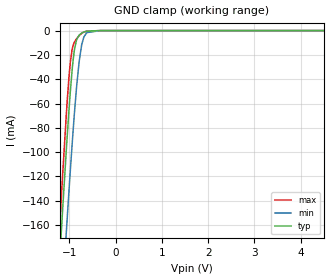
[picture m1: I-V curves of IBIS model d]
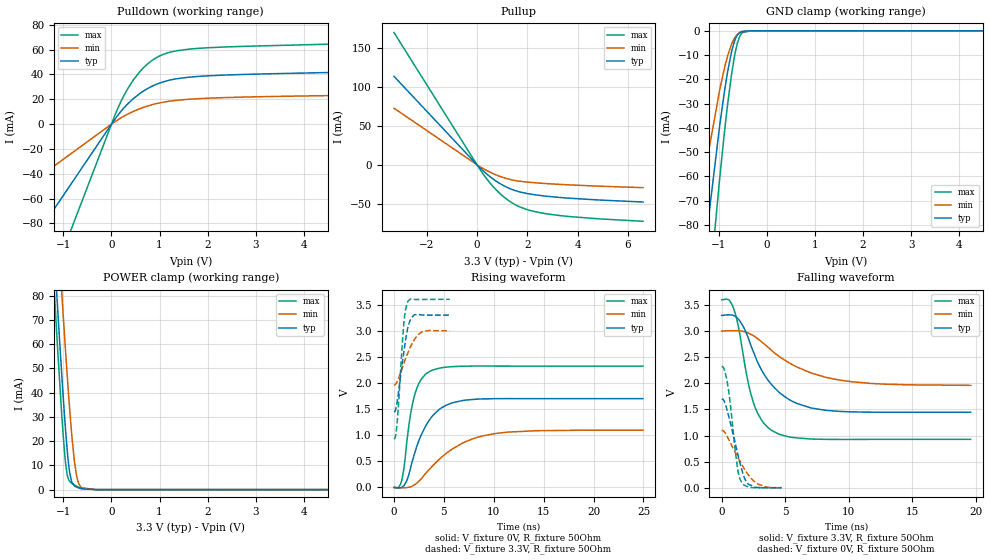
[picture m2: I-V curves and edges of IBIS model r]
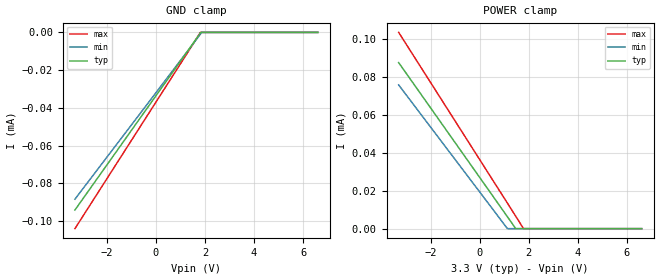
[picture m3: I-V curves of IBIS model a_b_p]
|Texas Instruments Incorporated
| 3.3V-supply RS-485
| Marketing part#   Digital Voltage Range   Package-type   #pins
| SN65HVD77DGK   3.0V-3.6V   VSSOP   8
| SN65HVD77DGKR   3.0V-3.6V   VSSOP   8
| SN65HVD77D   3.0V-3.6V   SOIC   8
| SN65HVD77DR   3.0V-3.6V   SOIC   8
[IBIS Ver]   4.1
[File name]   sn65hvd77.ibs
[File Rev]   1.0
[Date]   7/9/2014
[Source]
| Texas Instruments Incorporated.
| Analog-eLab Design Center, HPA
| 12500 TI Blvd
| Dallas, TX -75243
[Notes]   Revision History:
| Rev 1.0: 7/9/2014
| - Initial version of the model
| - Model generated from simulations in TISPICE
| - Model matched to SPICE simulation
| - C_comp although listed in numerical order of value are
|   obtained from varying PVT conditions. For PVT conditions for
|   each specific value refer the buffer description under
|   respective [Model]. IBIS model user is responsible for using
|   appropriate C_comp to simulate for Signal Integrity.
|* EXCEPTION:   *
|* - For model d, there is leakage current in the GND   *
|*   clamp I-V Table because of the pullup on pad.   *
|* - For models a_b_p and a_b_n, there is leakage current in the   *
|*   POWER clamp and GND clamp I-V Table because of the resistor   *
|*   network connected to pad.   *
[Disclaimer]
| This model is designed as an aid for customers of Texas Instruments.
| TI and its licensors and suppliers make no warranties, either expressed
| or implied, with respect to this  model, including the warranties of
| merchantability or fitness for a particular purpose. The model is
| provided solely on an "as is" basis. The entire risk as to its quality
| and performance is with the customer.
[Copyright]
(C) Copyright 2014 Texas Instruments Incorporated.All rights reserved.
|   SN65HVD77DGK
[Component]   SN65HVD77DGK
[Manufacturer]   TI
[Package]   |8 VSSOP  -  DGK package
|   typ   min   max
R_pkg   0.2   0.16   0.24
L_pkg   1.5nH   1.2nH   1.8nH
C_pkg   0.4pF   0.32pF   0.48pF
[Pin]  signal_name   model_name   R_pin   L_pin   C_pin
1   VCC   power   NA   NA   NA
2   R   r   NA   NA   NA
3   D   d   NA   NA   NA
4   GND   gnd   NA   NA   NA
5   Y   y_z_p   NA   NA   NA
6   Z   y_z_n   NA   NA   NA
7   B   a_b_n   NA   NA   NA
8   A   a_b_p   NA   NA   NA
[Diff_pin]   inv_pin   vdiff   tdelay_typ   tdelay_min   tdelay_max
5   6   0   NA   NA   NA
8   7   0.2V   NA   NA   NA
|   SN65HVD77D
[Component]   SN65HVD77D
[Manufacturer]   TI
[Package]   |8 SOIC  -  D package
|   typ   min   max
R_pkg   0.2   0.16   0.24
L_pkg   1.5nH   1.2nH   1.8nH
C_pkg   0.4pF   0.32pF   0.48pF
[Pin]  signal_name   model_name   R_pin   L_pin   C_pin
1   VCC   power   NA   NA   NA
2   R   r   NA   NA   NA
3   D   d   NA   NA   NA
4   GND   gnd   NA   NA   NA
5   Y   y_z_p   NA   NA   NA
6   Z   y_z_n   NA   NA   NA
7   B   a_b_n   NA   NA   NA
8   A   a_b_p   NA   NA   NA
[Diff_pin]   inv_pin   vdiff   tdelay_typ   tdelay_min   tdelay_max
5   6   0   NA   NA   NA
8   7   0.2V   NA   NA   NA
| Models and submodels in the file (6): d (Input), r (3-state), a_b_p (Input), a_b_n (Input), y_z_p (Output), y_z_n (Output)
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|   d Model
[Model]   d
Model_type   Input
Vinl = 0.8
Vinh = 2
|   typ   min   max
|   (nom PVT)   (fast PVT)   (slow PVT)
|Average
C_comp   2.191e-12   2.010e-12   2.367e-12
| Where nom  PVT is Nominal Process, 3.3V, 27C
|   Fast PVT is Strong Process,  3.6V, -40C
|   Slow PVT is Weak Process,   3V, 150C
[Voltage Range]   3.3   3   3.6
|Ambient Temperature   25   125   -40
|Junction Temperature
[Temperature Range]   27   150   -40
[Power Clamp Reference]   3.3   3   3.6
[GND Clamp Reference]   0   0   0
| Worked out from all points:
|   GND clamp passes 1 mA (typ) near -0.67 V on its own axis
[GND Clamp]
|   Voltage   I(typ)   I(min)   I(max)
-3.3V     -1.706A    -1.709A    -1.74A
-1.33V    -268.5mA   -332.2mA   -244.5mA
-1.176V   -166.3mA   -233.3mA   -138.2mA
-1.064V   -96.82mA   -164.4mA   -67.68mA
-980.1mV  -50.33mA   -115.2mA   -26.33mA
-945.6mV  -34.42mA   -96.08mA   -16.53mA
-891mV    -15.86mA   -67.76mA   -9.449mA
-789mV    -3.689mA   -25.45mA   -4.166mA
-735mV    -2.045mA   -11.84mA   -2.349mA
-686.4mV  -1.145mA   -5.17mA    -1.213mA
-330mV    -2.214uA   -10.64uA   -3.071uA
6.6V      0A         0A         0A
[POWER Clamp]
|   Voltage   I(typ)   I(min)   I(max)
-3.3V     0A         0A         0A
0V        0A         0A         0A
6.6V      0A         0A         0A
|   r Model
[Model]   r
Model_type   3-state
Polarity   Non-Inverting
Vmeas = 1.65
Vref = 0
Cref = 2pF
Rref = 100
|   typ   min   max
|   (nom PVT)   (fast PVT)   (slow PVT)
C_comp   1.738e-12   1.292e-12   1.903e-12
| Where nom  PVT is Nominal Process, 3.3V, 27C
|   Fast PVT is Strong Process,  3.6V, -40C
|   Slow PVT is Weak Process,   3V, 150C
[Voltage Range]   3.3   3   3.6
|Ambient Temperature   25   125   -40
|Junction Temperature
[Temperature Range]   27   150   -40
[Pullup Reference]   3.3   3   3.6
[Pulldown Reference]   0   0   0
[Power Clamp Reference]   3.3   3   3.6
[GND Clamp Reference]   0   0   0
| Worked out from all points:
|   slope of the pulldown table from 0 to 0.495 V, typ, clamps not added: 22.7 ohm
|   slope of the pullup table from 0 to 0.495 V, typ, clamps not added: 33.6 ohm
|   GND clamp passes 1 mA (typ) near -0.58 V on its own axis
|   POWER clamp passes 1 mA (typ) near -0.72 V on its own axis
|   falling waveform, V_fixture 3.3V, R_fixture 50Ohm: 20-80 % time 2.58ns typ, 4.29ns min, 1.43ns max; typ from 3.3 V to 1.45 V
|   rising waveform, V_fixture 0V, R_fixture 50Ohm: 20-80 % time 2.19ns typ, 4.23ns min, 1.16ns max; typ from 0 V to 1.7 V
|   rising waveform, V_fixture 3.3V, R_fixture 50Ohm: 20-80 % time 809ps typ, 1.31ns min, 547ps max; typ from 1.45 V to 3.3 V
|   falling waveform, V_fixture 0V, R_fixture 50Ohm: 20-80 % time 1.03ns typ, 1.54ns min, 651ps max; typ from 1.7 V to 0.001 V
[Pulldown]
|   Voltage   I(typ)   I(min)   I(max)
-3.3V     -189.2mA   -93.21mA   -333.8mA
-150mV    -8.602mA   -4.237mA   -15.17mA
81mV      4.532mA    2.189mA    8.151mA
206.4mV   10.74mA    5.253mA    19.04mA
447.6mV   20.3mA     10.13mA    35.16mA
746.4mV   28.56mA    14.54mA    48.37mA
1.046V    33.72mA    17.44mA    55.75mA
1.353V    36.55mA    19.18mA    59.09mA
1.821V    38.48mA    20.55mA    61.09mA
5.581V    43.1mA     23.86mA    66.87mA
6.136V    45.46mA    24.99mA    71.1mA
6.6V      49.39mA    26.86mA    78.08mA
[GND Clamp]
|   Voltage   I(typ)   I(min)   I(max)
-3.3V     -709.9mA   -433.2mA   -924.2mA
-1.468V   -124.3mA   -82.99mA   -167.5mA
-1.227V   -79.57mA   -51.57mA   -112.9mA
-1.198V   -74.42mA   -48.04mA   -106.4mA
-983.4mV  -39.11mA   -24.43mA   -60.91mA
-885mV    -25.16mA   -15.47mA   -41.95mA
-815.1mV  -16.54mA   -10.15mA   -29.8mA
-736.8mV  -8.691mA   -5.508mA   -18.1mA
-657mV    -3.351mA   -2.442mA   -8.683mA
-564.3mV  -653.4uA   -732.9uA   -2.153mA
-513.6mV  -211.6uA   -334.8uA   -709.7uA
6.6V      0A         0A         0A
[Pullup]
|   Voltage   I(typ)   I(min)   I(max)
-3.3V     113.5mA    72.59mA    169.7mA
159.6mV   -5.184mA   -3.23mA    -7.91mA
656.7mV   -18.69mA   -11.6mA    -28.54mA
1.128V    -27.96mA   -17.22mA   -42.86mA
1.445V    -32.34mA   -19.77mA   -49.86mA
1.731V    -35.11mA   -21.28mA   -54.48mA
2.183V    -37.94mA   -22.79mA   -59.24mA
2.721V    -40.22mA   -24.11mA   -62.73mA
3.633V    -42.86mA   -25.81mA   -66.37mA
6.6V      -47.83mA   -29.4mA    -72.58mA
[POWER Clamp]
|   Voltage   I(typ)   I(min)   I(max)
-3.3V     876.3mA    890.4mA    877.9mA
-1.278V   128.2mA    161.3mA    112.6mA
-1.14V    81.13mA    115.1mA    64.55mA
-1.033V   46.72mA    80.64mA    30.28mA
-950.4mV  23.21mA    55.47mA    10.04mA
-907.5mV  13.31mA    43.17mA    5.003mA
-867.9mV  6.78mA     32.54mA    3.359mA
-771mV    1.533mA    11.55mA    1.875mA
-722.7mV  983.9uA    5.305mA    1.349mA
-618mV    335.7uA    759.6uA    475.6uA
-330mV    645nA      5.334uA    223.6nA
6.6V      0A         0A         0A
[Ramp]
R_load = 50
|   typ   min   max
dV/dt_r   1.01934/2.19097e-09   0.65796/4.21113e-09   1.39293/1.15284e-09
dV/dt_f   1.11245/2.5768e-09   0.624322/4.26931e-09   1.60346/1.42875e-09
[Falling Waveform]
V_fixture = 3.3V
V_fixture_min = 3V
V_fixture_max = 3.6V
R_fixture = 50Ohm
|   Time   V(typ)   V(min)   V(max)
0s        3.3V       3V         3.6V
585ps     3.31V      3.008V     3.597V
1.025ns   3.289V     3.007V     3.371V
2.085ns   2.872V     2.963V     2.014V
2.645ns   2.512V     2.888V     1.529V
3.285ns   2.193V     2.765V     1.244V
4.15ns    1.915V     2.582V     1.069V
5.955ns   1.612V     2.308V     953.7mV
9.03ns    1.467V     2.073V     925.6mV
19.6ns    1.446V     1.961V     927.6mV
[Rising Waveform]
V_fixture = 0V
V_fixture_min = 0V
V_fixture_max = 0V
R_fixture = 50Ohm
|   Time   V(typ)   V(min)   V(max)
0s        2.154nV    302nV      347.2pV
475ps     -7.446mV   -5.111mV   4.066mV
800ps     3.571mV    -5.552mV   154.8mV
1.61ns    330.5mV    9.326mV    1.341V
2.15ns    703.9mV    62.45mV    1.818V
2.765ns   1.019V     172.1mV    2.08V
3.78ns    1.351V     394.7mV    2.239V
5.855ns   1.62V      737.5mV    2.312V
10.11ns   1.699V     1.03V      2.323V
24.95ns   1.699V     1.097V     2.322V
[Rising Waveform]
V_fixture = 3.3V
V_fixture_min = 3V
V_fixture_max = 3.6V
R_fixture = 50Ohm
|   Time   V(typ)   V(min)   V(max)
0s        1.446V     1.959V     927.6mV
165ps     1.49V      1.975V     996mV
330ps     1.653V     2.031V     1.273V
995ps     2.607V     2.379V     3.16V
1.18ns    2.839V     2.473V     3.423V
1.355ns   3.028V     2.558V     3.542V
1.57ns    3.175V     2.655V     3.592V
1.92ns    3.284V     2.791V     3.6V
2.72ns    3.304V     2.967V     3.597V
5.595ns   3.299V     2.998V     3.6V
[Falling Waveform]
V_fixture = 0V
V_fixture_min = 0V
V_fixture_max = 0V
R_fixture = 50Ohm
|   Time   V(typ)   V(min)   V(max)
0s        1.699V     1.097V     2.322V
225ps     1.641V     1.065V     2.245V
490ps     1.428V     953.8mV    1.945V
685ps     1.239V     859.2mV    1.589V
1.255ns   651.8mV    589mV      354.3mV
1.47ns    440.5mV    493.2mV    147.9mV
1.845ns   159.1mV    336.4mV    43.14mV
2.195ns   53.63mV    216.7mV    10.44mV
3.17ns    -300.2uV   41.79mV    719.7uV
4.72ns    855.9uV    -2.271mV   348.8uV
|   a_b Model
[Model]   a_b_p
Model_type   Input
Vinl = 0.8
Vinh = 2
|   typ   min   max
|   (nom PVT)   (fast PVT)   (slow PVT)
|Average
C_comp   3.329e-12   3.222e-12   3.479e-12
| Where nom  PVT is Nominal Process, 3.3V, 27C
|   Fast PVT is Strong Process,  3.6V, -40C
|   Slow PVT is Weak Process,   3V, 150C
[Voltage Range]   3.3   3   3.6
|Ambient Temperature   25   125   -40
|Junction Temperature
[Temperature Range]   27   150   -40
[Power Clamp Reference]   3.3   3   3.6
[GND Clamp Reference]   0   0   0
[GND Clamp]
|   Voltage   I(typ)   I(min)   I(max)
-3.3V     -94.21uA   -88.46uA   -104.1uA
1.812V    -325.9nA   -970.2nA   -10.18nA
1.872V    0A         0A         0A
6.6V      0A         0A         0A
[POWER Clamp]
|   Voltage   I(typ)   I(min)   I(max)
-3.3V     87.61uA    75.84uA    103.6uA
1.131V    6.277uA    0A         13.47uA
1.468V    35.36nA    0A         6.584uA
1.787V    0A         0A         14.67nA
6.6V      0A         0A         0A
